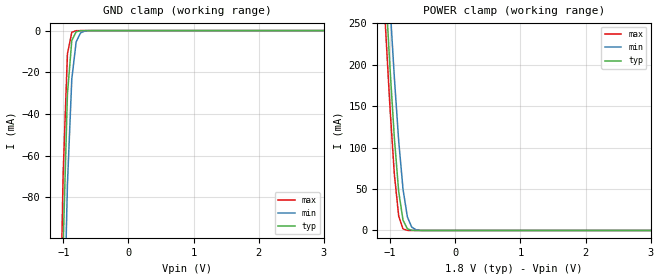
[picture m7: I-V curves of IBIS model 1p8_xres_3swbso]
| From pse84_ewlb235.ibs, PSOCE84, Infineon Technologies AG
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[Model] 1p8_xres_3swbso
Model_type Input
Vinl  =  0.54
Vinh  =  1.26
| Capacitance   typ   min   max
C_comp   5.38278e-13 5.24637e-13 5.54090e-13
| Variables   typ   min   max
[GND Clamp Reference]   0   0   0
[POWER Clamp Reference]   1.8   1.66   1.89
[Pulldown Reference]   0   0   0
[Pullup Reference]   1.8   1.66   1.89
[Temperature Range]   25   125   -40
[Voltage Range]   1.8   1.66   1.89
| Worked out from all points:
|   GND clamp passes 1 mA (typ) near -0.81 V on its own axis
|   POWER clamp passes 1 mA (typ) near -0.70 V on its own axis
[GND Clamp]
| Voltage   I(typ)   I(min)   I(max)
-1.405V   -942.6mA   -981.9mA   -923mA
-1.07V    -218.9mA   -278mA     -182.8mA
-1.003V   -104.9mA   -162.7mA   -69.97mA
-936.6mV  -30.48mA   -73.83mA   -11.23mA
-869.7mV  -4.814mA   -23.33mA   -832.9uA
-802.8mV  -581.2uA   -5.445mA   -52.93uA
-735.9mV  -66.75uA   -1.122mA   -3.324uA
-669mV    -7.618uA   -222.9uA   -208.7nA
3.6V      0A         0A         0A
[POWER Clamp]
| Voltage   I(typ)   I(min)   I(max)
-1.472V   892.3mA    954.3mA    855.4mA
-1.07V    290.4mA    365.7mA    243mA
-1.003V   196.8mA    272.6mA    148.8mA
-936.6mV  112.3mA    185.3mA    68.47mA
-869.7mV  47.11mA    108.4mA    17.57mA
-802.8mV  12.44mA    49.7mA     1.84mA
-735.9mV  1.986mA    16.35mA    126.5uA
-669mV    240.4uA    3.968mA    8.262uA
-602.1mV  27.35uA    809.2uA    536.8nA
-401.4mV  38.03nA    5.437uA    153.8pA
3.6V      0A         0A         0A
